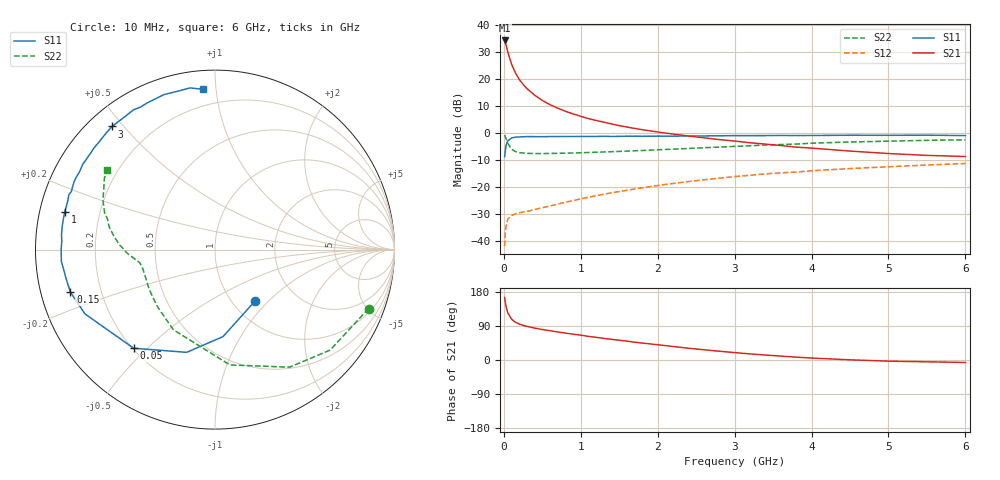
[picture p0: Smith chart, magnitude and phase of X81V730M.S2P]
! SIEMENS Small Signal Semiconductors
! BFP136W
! Si NPN RF Bipolar Junction Transistor in SOT343
! VCE = 1.75 V  IC = 30 mA
! Common Emitter S-Parameters:  September  1994
# GHz  S  MA  R  50
!  f  S11  S21  S12  S22
! GHz  MAG  ANG  MAG  ANG  MAG  ANG  MAG  ANG
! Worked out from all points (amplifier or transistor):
!   40 points, 10 MHz to 6 GHz, reference 50 ohm
!   highest |S21| = 34.4 dB at 10 MHz (marker M1)
!   |S21| within 3 dB of that: start of sweep to 40.09 MHz
!   unconditionally stable (mu >= 1): 728.8 MHz to 2.809 GHz
!   at 200 MHz: K = 0.43, MSG = 24.8 dB, |S12| = -29.7 dB
!   at 1.5 GHz: K = 1.15, MAG = 9.9 dB, |S12| = -21.7 dB
!   at 6 GHz: K = 0.98, MSG = 1.3 dB, |S12| = -11.3 dB
!   S11 on the Smith chart (normalised r, x): 10 MHz: 1.26, -0.84; 50 MHz: 0.20, -0.46; 150 MHz: 0.09, -0.14; 1 GHz: 0.07, +0.12; 3 GHz: 0.07, +0.47; 6 GHz: 0.10, +0.92
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0.01  0.3632 -52.3  52.49 164.9  0.0079 75.1  0.9165 -21.0
0.02  0.4867 -84.7  47.47 151.3  0.0144 63.9  0.8515 -41.1
0.03  0.5937 -105.4  42.54 140.4  0.0193 53.9  0.7758 -57.6
0.05  0.7123 -129.5  32.55 125.3  0.0248 40.7  0.6481 -82.6
0.1  0.8083 -153.7  19.04 107.9  0.0295 29.5  0.5032 -117.5
0.15  0.84 -163.6  13.13 99.8  0.0315 27.4  0.4524 -134.8
0.2  0.8456 -169.2  9.916 94.9  0.0329 27.7  0.4334 -144.7
0.25  0.8514 -173.0  8.013 91.5  0.0341 29.0  0.4249 -151.1
0.3  0.8585 -175.6  6.709 88.8  0.0349 30.9  0.4186 -155.3
0.4  0.8571 179.9  5.061 84.2  0.0379 34.4  0.4162 -160.9
0.5  0.855 176.7  4.035 80.4  0.041 37.9  0.4157 -164.3
0.6  0.8592 174.4  3.363 77.3  0.0441 41.1  0.4173 -166.4
0.8  0.8615 169.5  2.537 71.1  0.0517 46.2  0.4229 -169.0
1  0.8631 165.8  2.044 65.6  0.0598 49.4  0.43 -170.7
1.1  0.8629 163.1  1.854 62.2  0.0639 50.7  0.4349 -171.4
1.5  0.8668 156.3  1.373 52.2  0.0819 53.6  0.455 -173.9
2.2  0.8761 143.8  0.957 35.7  0.1154 52.7  0.5012 -179.1
3  0.8944 129.9  0.709 19.5  0.1548 47.6  0.5646 173.0
3.2  0.8935 126.5  0.66 16.1  0.1641 46.1  0.5797 170.8
4.5  0.9093 108.2  0.462 0.5  0.2185 34.5  0.6818 156.3
5.5  0.9116 98.8  0.384 -4.8  0.2542 26.3  0.7318 147.4
6  0.8959 94.4  0.366 -6.5  0.2711 21.8  0.7488 143.7
